(* 	
	Program Name: 	ACS_CMD_HOME
	Purpose:		Copy Home Command to ACS Drive Output Command Register
	When Executed:	Executes homing profile action defined in TMI
*)
PROGRAM ACS_CMD_HOME
VAR_IN_OUT
	Axis:ACS_DRIVE_TYPE;
END_VAR
VAR
	_command:	USINT	:= ACS_COMMANDS.HOME;
END_VAR

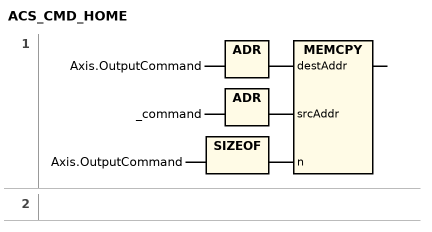
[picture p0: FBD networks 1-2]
// NETWORK 1
MEMCPY(destAddr := ADR(Axis.OutputCommand), srcAddr := ADR(_command), n := SIZEOF(Axis.OutputCommand));

// NETWORK 2

END_PROGRAM
